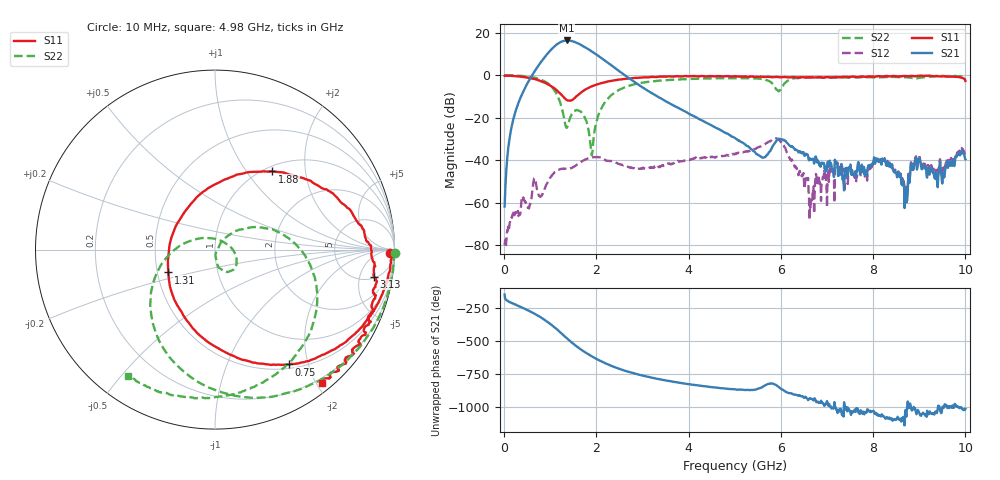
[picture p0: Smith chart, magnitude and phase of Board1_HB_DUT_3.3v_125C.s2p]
! Created Tue May 27 14:57:15 2025
# hz S ma R 50
! 2 Port Network Data from SP1.SP block
! freq  magS11  angS11  magS21  angS21  magS12  angS12  magS22  angS22
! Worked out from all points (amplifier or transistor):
!   1000 points, 10 MHz to 10 GHz, reference 50 ohm
!   highest |S21| = 16.4 dB at 1.36 GHz (marker M1)
!   |S21| within 3 dB of that: 1.08 GHz to 1.741 GHz (661.3 MHz wide, 46.9 % of centre)
!   unconditionally stable (mu >= 1): 16.24 MHz to 47.12 MHz; 51.69 MHz to end of sweep
!   at 1.67 GHz: K = 8.80, MAG = 15.1 dB, |S12| = -40.8 dB
!   at 5.01 GHz: K = 23.43, MAG = -13.0 dB, |S12| = -37.0 dB
!   at 10 GHz: K = 498.58, MAG = -30.9 dB, |S12| = -37.8 dB
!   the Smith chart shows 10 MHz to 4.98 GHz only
!   S11 on the Smith chart (normalised r, x): 10 MHz: 53, -33; 750 MHz: 0.56, -1.70; 1.31 GHz: 0.57, -0.16; 1.88 GHz: 1.08, +1.33; 3.13 GHz: 5, -8; 4.98 GHz: 0.13, -2.08
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1e7  0.9731 -1.0  0.0008064 -144.7  9.703e-05 101.3  1.004 -0.9
2.2e8  0.9633 -15.2  0.1117 141.3  0.0005029 83.8  0.9896 -20.3
7.5e8  0.7615 -57.2  1.73 50.8  0.001489 72.1  0.8279 -80.9
9.3e8  0.6328 -76.1  3.147 10.1  0.002792 118.3  0.6664 -110.3
1.09e9  0.4933 -98.6  4.802 -33.2  0.005081 101.2  0.4439 -143.9
1.19e9  0.394 -118.1  5.817 -63.5  0.005951 87.6  0.2718 -170.9
1.31e9  0.2898 -154.0  6.561 -101.9  0.006258 75.5  0.08506 129.9
1.36e9  0.2597 -174.7  6.645 -117.7  0.006255 73.1  0.05846 63.3
1.51e9  0.279 122.1  6.231 -162.5  0.00694 73.5  0.1388 -30.0
1.68e9  0.4021 79.9  5.127 153.3  0.009262 66.0  0.132 -65.8
1.88e9  0.5388 54.0  3.786 109.1  0.01134 45.6  0.01957 -75.4
2.24e9  0.7106 27.5  2.009 45.5  0.009665 13.1  0.2745 27.2
2.6e9  0.8233 9.5  1.035 -2.3  0.007671 1.8  0.5146 -5.8
3.13e9  0.8983 -9.6  0.4227 -51.7  0.00649 13.7  0.7042 -41.6
3.34e9  0.9202 -15.7  0.3089 -67.2  0.007102 9.7  0.7445 -53.8
4.98e9  0.9515 -51.2  0.03458 -145.2  0.01401 -11.1  0.8538 -124.7
5.01e9  0.9575 -51.9  0.03284 -146.8  0.01405 -11.9  0.8552 -125.8
5.94e9  0.9087 -71.5  0.0303 -124.5  0.03112 -97.5  0.4377 -152.1
6.67e9  0.8977 -92.0  0.01035 140.9  0.001176 129.9  0.9039 -157.5
8.34e9  0.9424 -133.8  0.007105 -8.5  0.007481 -13.5  0.913 166.8
8.7e9  0.9694 -140.3  0.001734 56.0  0.002126 52.3  0.897 160.0
1e10  0.7378 -161.3  0.01048 66.2  0.01281 62.7  0.8404 151.9
